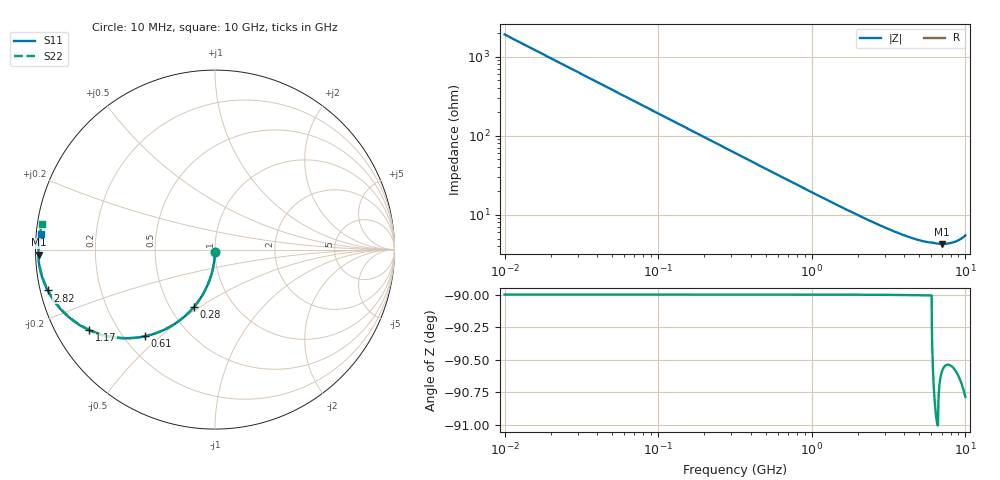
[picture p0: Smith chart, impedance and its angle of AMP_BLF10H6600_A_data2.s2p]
! Created Tue Feb  9 12:08:14 2010
# ghz S ma R 50
! 2 Port Network Data from SP1.SP block
! freq  magS11  angS11  magS21  angS21  magS12  angS12  magS22  angS22
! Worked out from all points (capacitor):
!   1000 points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, 10 MHz to 10 GHz, reference 50 ohm
!   read as one part in shunt: C = 8.34 pF near 60 MHz
!   lowest |Z| = 4.27 ohm at 6.99 GHz (marker M1)
!   S11 on the Smith chart (normalised r, x): 10 MHz: 1.00, -0.03; 280 MHz: 0.65, -0.47; 610 MHz: 0.28, -0.45; 1.17 GHz: 0.10, -0.29; 2.82 GHz: 0.02, -0.12; 10 GHz: 0.01, +0.05
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0.01  0.01302 -90.8  0.9999 -0.8  0.9999 -0.8  0.01302 -90.8
0.04  0.05202 -93.0  0.9986 -3.0  0.9986 -3.0  0.05202 -93.0
0.07  0.09078 -95.3  0.9959 -5.3  0.9959 -5.3  0.09078 -95.3
0.09  0.1164 -96.8  0.9932 -6.8  0.9932 -6.8  0.1164 -96.8
0.11  0.1418 -98.2  0.9899 -8.3  0.9899 -8.3  0.1418 -98.3
0.14  0.1793 -100.4  0.9838 -10.5  0.9838 -10.5  0.1793 -100.5
0.18  0.2282 -103.3  0.9736 -13.4  0.9736 -13.4  0.2282 -103.4
0.28  0.3424 -110.3  0.9396 -20.3  0.9396 -20.3  0.3424 -110.3
0.42  0.4793 -119.0  0.8777 -29.0  0.8777 -29.0  0.4793 -119.1
0.61  0.6207 -128.9  0.784 -39.0  0.784 -39.0  0.6207 -129.0
0.88  0.7512 -139.4  0.66 -49.5  0.66 -49.5  0.7512 -139.6
1.17  0.833 -147.4  0.5533 -57.5  0.5533 -57.5  0.833 -147.7
1.41  0.8747 -152.2  0.4847 -62.4  0.4847 -62.4  0.8747 -152.5
1.68  0.9056 -156.4  0.4242 -66.5  0.4242 -66.5  0.9056 -156.7
2.17  0.9383 -161.7  0.3458 -71.9  0.3458 -71.9  0.9383 -162.2
2.82  0.96 -166.3  0.28 -76.6  0.28 -76.6  0.96 -166.9
3.34  0.9694 -168.9  0.2455 -79.3  0.2455 -79.3  0.9694 -169.6
5.01  0.9821 -174.2  0.1882 -84.8  0.1882 -84.8  0.9821 -175.4
6.67  0.983 -177.7  0.1695 -89.4  0.1695 -89.4  0.9831 -179.4
6.99  0.9837 -178.4  0.1693 -89.9  0.1693 -89.9  0.9838 179.8
8.34  0.9824 179.0  0.1772 -92.8  0.1772 -92.8  0.9824 176.6
10  0.9736 174.8  0.2154 -97.7  0.2154 -97.7  0.9735 171.5
